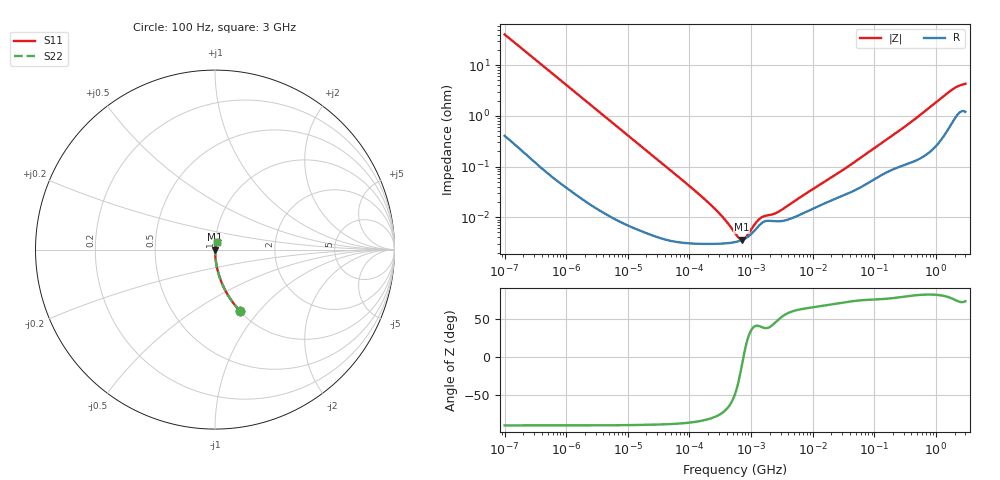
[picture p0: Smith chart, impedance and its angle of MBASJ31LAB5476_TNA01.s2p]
! MBASJ31LAB5476_TNA01  S-PARAMETER MODEL  ( Standard Model )
! Model Generated by TAIYO YUDEN Corporation (http://www.ty-top.com)
! Version 2.0
! TAIYO YUDEN Control No. 230906
! Copyright(c) 2012 TAIYO YUDEN CO.,LTD. All Rights Reserved.
! Product Description (link to TY-COMPAS)
! https://ds.yuden.co.jp/TYCOMPAS/or/detail?pn=MBASJ31LAB5476MTNA01&u=M
! Products Name : Multilayer Ceramic Capacitors
! Characteristics :
!  Capacitance : 47 [uF] , Rated Voltage : 6.3 [V] , TCC : X5R
!  Case Size : 3.2 x 1.6 / 0.126 x 0.063 [mm/inch] , Thickness : 1.6 / 0.063 [mm/inch]
!  (Conditions: Temperature = 25 [degC] , DC Bias Voltage = 0 [V])
! External Node Assignments :
!  1  o---| |---o  2
! GND o---------o GND
! Frequency Range : 100Hz  -  3GHz  [ 401 STEP ]
# MHZ S RI R 50
! Freq[MHz].  S11 Real  S11 Imag  S21 Real  S21 Imag  S12 Real  S12 Imag  S22 Real  S22 Imag
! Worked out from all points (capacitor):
!   401 points, 100 Hz to 3 GHz, reference 50 ohm
!   read as one part in series: C = 39.6 uF near 109 Hz
!   lowest |Z| = 3.6 mohm at 709.1 kHz (marker M1)
!   series resonance near 750.3 kHz, so ESL is about 1.1 nH
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0.0001  0.1414 -0.3435  0.8586 0.3435  0.8586 0.3435  0.1414 -0.3435
0.000114  0.1134 -0.3121  0.8866 0.3121  0.8866 0.3121  0.1134 -0.3121
0.000175  0.0523 -0.2179  0.9477 0.2179  0.9477 0.2179  0.0523 -0.2179
0.000348  0.0143 -0.1144  0.9857 0.1144  0.9857 0.1144  0.0143 -0.1144
0.000724  0.00365 -0.0559  0.9964 0.0559  0.9964 0.0559  0.00365 -0.0559
0.001788  0.00075 -0.0228  0.9992 0.0228  0.9992 0.0228  0.00075 -0.0228
0.031977  4.11e-05 -0.0013  1 0.0013  1 0.0013  4.11e-05 -0.0013
0.144239  3e-05 -0.000279  1 0.000279  1 0.000279  3e-05 -0.000279
0.341146  3.02e-05 -9.81e-05  1 9.81e-05  1 9.81e-05  3.02e-05 -9.81e-05
0.388167  3.06e-05 -7.98e-05  1 7.98e-05  1 7.98e-05  3.06e-05 -7.98e-05
0.547723  3.23e-05 -3.64e-05  1 3.64e-05  1 3.64e-05  3.23e-05 -3.64e-05
0.709116  3.54e-05 -6.45e-06  1 6.45e-06  1 6.45e-06  3.54e-05 -6.45e-06
1.411895  7.27e-05 6.22e-05  0.9999 -6.22e-05  0.9999 -6.22e-05  7.27e-05 6.22e-05
2.366551  8.34e-05 8.18e-05  0.9999 -8.18e-05  0.9999 -8.18e-05  8.34e-05 8.18e-05
3.198641  8.43e-05 0.000114  0.9999 -0.000114  0.9999 -0.000114  8.43e-05 0.000114
9.794414  0.000145 0.000319  0.9999 -0.000319  0.9999 -0.000319  0.000145 0.000319
31.31008  0.000269 0.000819  0.9997 -0.000819  0.9997 -0.000819  0.000269 0.000819
175.1444  0.000826 0.0036  0.9992 -0.0036  0.9992 -0.0036  0.000826 0.0036
414.2403  0.00128 0.00778  0.9987 -0.00778  0.9987 -0.00778  0.00128 0.00778
1714.41  0.00727 0.03  0.9927 -0.03  0.9927 -0.03  0.00727 0.03
2219.584  0.0116 0.0356  0.9884 -0.0356  0.9884 -0.0356  0.0116 0.0356
3000  0.0135 0.0401  0.9865 -0.0401  0.9865 -0.0401  0.0135 0.0401
